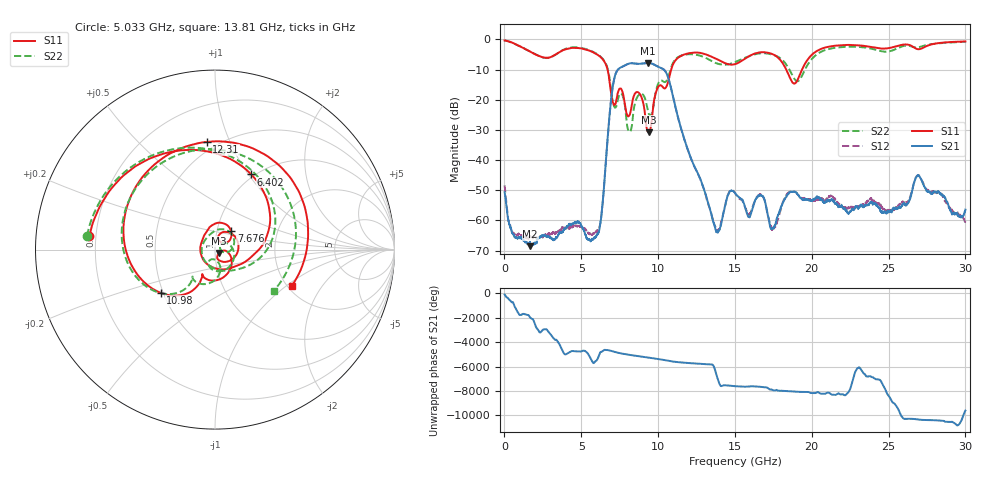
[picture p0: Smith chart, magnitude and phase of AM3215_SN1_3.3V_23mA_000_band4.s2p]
!Agilent Technologies,E8364B,MY43040894,A.07.50.67
!Agilent E8364B: A.07.50.67
!Date: Tuesday, May 25, 2021 15:16:08
!Correction: S11(Full 2 Port(1,2))
!S21(Full 2 Port(1,2))
!S12(Full 2 Port(1,2))
!S22(Full 2 Port(1,2))
!S2P File: Measurements: S11, S21, S12, S22:
# Hz S  dB  R 50
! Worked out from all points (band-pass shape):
!   6401 points, 10 MHz to 30 GHz, reference 50 ohm
!   highest |S21| = -7.80 dB at 9.326 GHz (marker M1); lowest = -68.5 dB at 1.669 GHz (marker M2)
!   |S21| within 3 dB of the highest: 7.288 GHz to 10.5 GHz (3.211 GHz wide, 36.1 % of centre)
!   lowest |S11| = -30.9 dB at 9.387 GHz (marker M3), VSWR 1.06, Z = 52.1 - j2.01 ohm
!   |S11| at or under -10 dB: 6.708 GHz to 10.85 GHz (4.145 GHz wide, 47.2 % of centre); 18.34 GHz to 19.37 GHz (1.035 GHz wide, 5.49 % of centre)
!   |S22| runs from -30.7 to -0.4 dB; largest |S21 - S12| = 0.0052
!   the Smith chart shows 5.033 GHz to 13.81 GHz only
!   S11 on the Smith chart (normalised r, x): 5.033 GHz: 0.17, +0.05; 6.402 GHz: 0.96, +1.03; 7.676 GHz: 1.17, +0.24; 10.98 GHz: 0.48, -0.27; 12.31 GHz: 0.44, +0.82; 13.81 GHz: 2.11, -1.09
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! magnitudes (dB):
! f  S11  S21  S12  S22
! 10 MHz  -0.4  -50.6  -48.4  -0.4
! 1.669 GHz  -4.1  -68.5  -65.4  -4.0
! 5.01 GHz  -3.0  -61.8  -62.1  -2.9
! 5.033 GHz  -3.0  -62.1  -62.2  -2.9
! 6.402 GHz  -6.7  -53.8  -53.8  -6.5
! 7.039 GHz  -20.6  -16.1  -16.1  -20.4
! 7.676 GHz  -17.3  -9.0  -9.1  -18.5
! 8.126 GHz  -25.3  -8.0  -8.0  -30.7
! 8.735 GHz  -17.7  -8.1  -8.1  -18.5
! 9.326 GHz  -30.6  -7.8  -7.8  -23.4
! 9.387 GHz  -30.9  -7.8  -7.8  -24.6
! 10.01 GHz  -15.8  -9.1  -9.1  -14.6
! 10.98 GHz  -8.2  -19.0  -19.1  -7.7
! 12.31 GHz  -4.4  -41.5  -41.6  -5.0
! 13.81 GHz  -6.5  -63.9  -63.1  -8.0
! 15.01 GHz  -8.2  -50.9  -50.8  -7.5
! 17.49 GHz  -5.0  -62.4  -63.2  -5.1
! 18.86 GHz  -14.7  -50.5  -50.5  -13.0
! 20 GHz  -5.1  -53.5  -53.4  -6.5
! 25 GHz  -2.9  -57.3  -56.7  -4.0
! 26.94 GHz  -3.3  -45.1  -45.1  -2.6
! 30 GHz  -0.7  -56.4  -60.6  -0.8
